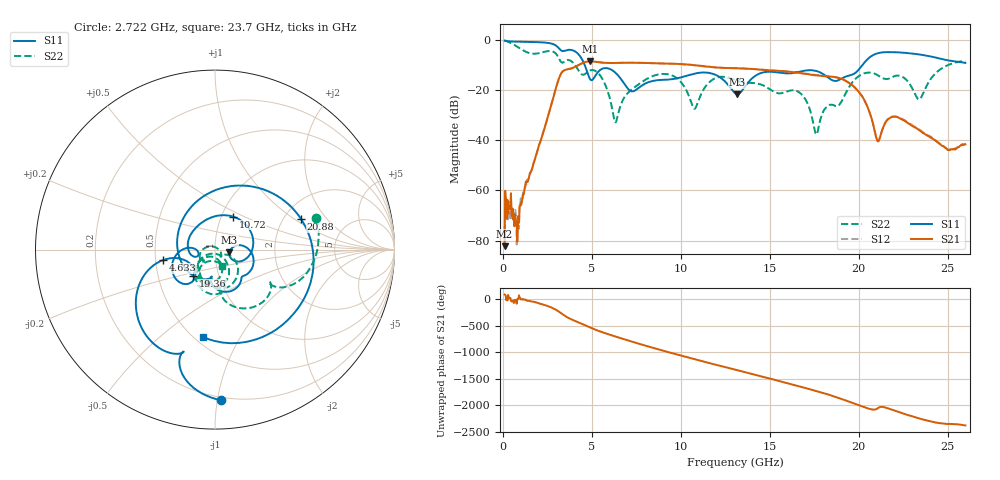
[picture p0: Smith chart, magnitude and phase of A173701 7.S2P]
!  2-Port S-parameters saved by WinCal
! VAR MeasName=S-Parameters (CALIBRATED_DATA) read from VNA (N5245A)
! VAR MeasDate=2017-6-7 10:28:51
! VAR NAME=A173701 7
! VAR FILENAME=A173701 7.S2P
! VAR DATE=2017-6-7 10:28:51
! VAR PHYS_PORTS=1,2
# Hz S DB R 50
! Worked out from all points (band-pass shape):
!   801 points, 100 MHz to 26 GHz, reference 50 ohm
!   highest |S21| = -8.59 dB at 4.924 GHz (marker M1); lowest = -82.2 dB at 100 MHz (marker M2)
!   |S21| within 3 dB of the highest: 3.766 GHz to 13.86 GHz (10.09 GHz wide, 115 % of centre)
!   lowest |S11| = -21.7 dB at 13.18 GHz (marker M3), VSWR 1.18, Z = 58.7 - j1.89 ohm
!   |S11| at or under -10 dB: 4.598 GHz to 20.22 GHz (15.62 GHz wide, 126 % of centre)
!   |S22| runs from -37.7 to -0.3 dB; largest |S21 - S12| = 0.0049
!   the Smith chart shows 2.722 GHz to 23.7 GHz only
!   S11 on the Smith chart (normalised r, x): 2.722 GHz: 0.18, -1.03; 4.633 GHz: 0.55, -0.07; 10.72 GHz: 1.13, +0.44; 19.36 GHz: 0.76, -0.23; 20.88 GHz: 2.47, +1.14; 23.7 GHz: 0.55, -0.70
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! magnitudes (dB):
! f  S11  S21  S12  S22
! 100 MHz  -0.3  -82.2  -80.2  -0.3
! 261.9 MHz  -0.6  -63.8  -63.7  -0.7
! 779.9 MHz  -0.8  -72.7  -81.5  -2.7
! 2.722 GHz  -1.5  -25.9  -25.9  -4.6
! 3.337 GHz  -4.5  -12.8  -12.8  -9.1
! 4.438 GHz  -7.6  -9.4  -9.4  -13.8
! 4.633 GHz  -10.6  -8.9  -8.9  -13.6
! 4.924 GHz  -15.9  -8.6  -8.6  -12.2
! 6.348 GHz  -13.3  -9.3  -9.2  -32.9
! 7.255 GHz  -20.5  -9.2  -9.1  -19.7
! 8.744 GHz  -16.1  -9.4  -9.4  -13.8
! 10.72 GHz  -13.6  -10.1  -10.1  -27.2
! 13.05 GHz  -21.3  -11.3  -11.3  -16.1
! 13.18 GHz  -21.7  -11.4  -11.4  -16.4
! 16.58 GHz  -12.9  -13.1  -13.1  -20.6
! 17.39 GHz  -12.2  -14.0  -13.9  -31.3
! 17.65 GHz  -12.5  -14.2  -14.1  -37.6
! 19.36 GHz  -14.5  -16.8  -16.7  -20.1
! 20.88 GHz  -5.9  -35.7  -35.8  -13.5
! 21.69 GHz  -4.9  -31.4  -31.3  -15.5
! 23.7 GHz  -6.2  -37.5  -37.2  -20.2
! 26 GHz  -9.2  -41.7  -41.6  -8.6
